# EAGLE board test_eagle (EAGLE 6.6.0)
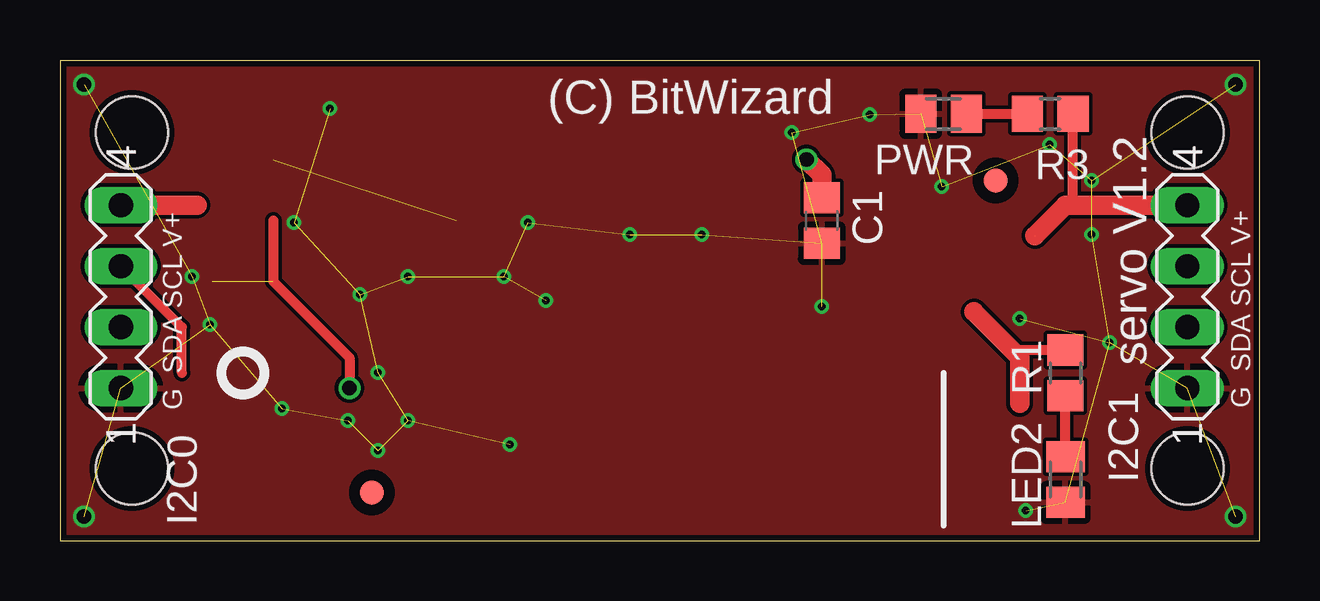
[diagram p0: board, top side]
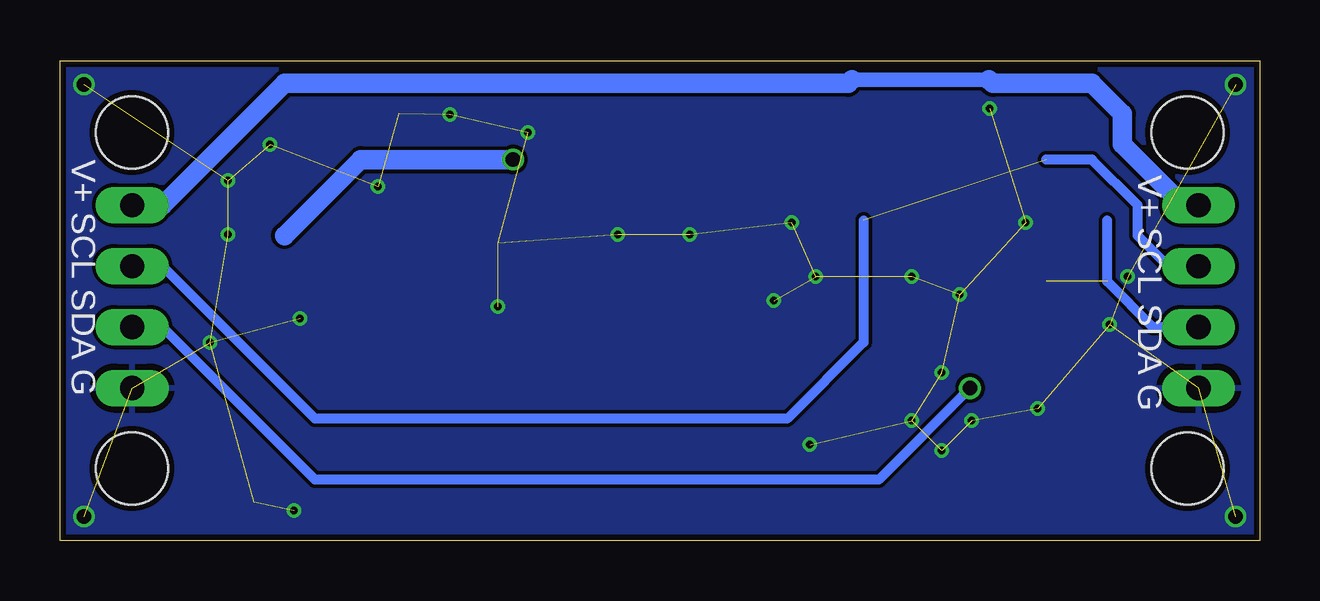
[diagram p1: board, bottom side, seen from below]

Size 50 x 20 mm. Coordinates in mm from the lower left corner, seen from the top.
Outline: 0,0 50,0 50,20 0,20 0,0
Copper layers (1*16): Top 0.035mm / dielectric 1.5mm / Bottom 0.035mm
Design rules "Fusion_eagle_rule_v1.1": minimum track width 6mil, minimum drill 12mil, track to track 6mil, track to pad 6mil, pad to pad 6mil, via to via 6mil, smd to smd 0mil, copper to edge 10mil, drill to drill 10mil, minimum pad ring 7mil, minimum via ring 6mil, stop-mask expansion 2mil, vias tented up to drill 100mil, thermal gap 10mil

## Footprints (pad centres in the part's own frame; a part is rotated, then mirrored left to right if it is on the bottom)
FID1 = smd 1 x 1: P$1 0,0
C0805 = smd 1.3 x 1.5: 1 -0.95,0; 2 0.95,0
MA04-1 = drill 1.016 long: 1 -3.81,0; 2 -1.27,0; 3 1.27,0; 4 3.81,0
M0805 = smd 1.3 x 1.6: 1 -0.95,0; 2 0.95,0
R0805 = smd 1.3 x 1.5: 1 -0.95,0; 2 0.95,0
MOUNTING_HOLE = hole 3: 0,0

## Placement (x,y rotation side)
AFIT1  FIDUCIAL1  [FID1]  13,2 0 top
AFIT2  FIDUCIAL1  [FID1]  39,15 0 top
C1  100n  [C0805]  31.75,13.34 270 top
I2C0  [MA04-1]  2.54,10.16 90 top
I2C1  [MA04-1]  46.99,10.16 90 top
LED2  G  [M0805]  41.91,2.54 270 top
PWR  G  [M0805]  36.83,17.78 180 top
R1  47k  [R0805]  41.91,6.99 90 top
R3  47k  [R0805]  41.27,17.78 0 top
U$2  MOUNTING_HOLE  [MOUNTING_HOLE]  3,3 0 top
U$3  MOUNTING_HOLE  [MOUNTING_HOLE]  3,17 0 top
U$4  MOUNTING_HOLE  [MOUNTING_HOLE]  47,3 0 top
U$5  MOUNTING_HOLE  [MOUNTING_HOLE]  47,17 0 top

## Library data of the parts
AFIT1 AFIT2 U$2-U$5 = hdr_altera
C1 R1 R3 = rcl
I2C0 I2C1 = con-lstb; OC_FARNELL: unknown; OC_NEWARK: unknown
LED2 PWR = myled

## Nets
GND: C1.2 I2C0.1 I2C1.1 LED2.2 PWR.2
N$1: I2C0.2 I2C1.2
N$6: PWR.1 R3.1
N$13: I2C0.3 I2C1.3
N$14: R1.2
N$15: LED2.1 R1.1
VCC: C1.1 I2C0.4 I2C1.4 R3.2

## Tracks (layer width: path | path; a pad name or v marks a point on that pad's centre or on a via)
GND  (via drill 0.3, 0.61)  (35 unrouted)
  other vias: 1,19 1,1 49,1 49,19 12,5 13.25,3.75 14.5,5 13.25,7 9.25,5.5 12.5,10.25 19.5,13.25 20.25,10 18.5,11 23.75,12.75 26.75,12.75 11.25,18 5.5,11 6.25,9 14.5,11 9.75,13.25 18.75,4 31.75,9.75 30.5,17 33.75,17.75 36.75,14.75 41.25,16.5 43,15 43,12.75 40.25,1.25 43.75,8.25 40,9.25
  pour Top: 0,20 0,0 50,0 50,20
  pour Bottom: 0,20 50,20 50,0 0,0
N$1  (via drill 0.61)  (1 unrouted)
  Top 0.406: 8.89,13.34 8.89,10.79 12.06,7.62 v12.06,6.35
  Bottom 0.406: I2C0.2 4.45,8.89 6.35,10.79 6.35,13.34 | v12.06,6.35 15.88,2.54 39.37,2.54 45.72,8.89 I2C1.2
N$6
  Top 0.406: PWR.1 R3.1
N$13  (1 unrouted)
  Top 0.406: 5.08,6.99 5.08,8.89 I2C0.3
  Bottom 0.406: 16.51,13.34 16.51,8.26 19.68,5.08 39.37,5.08 45.72,11.43 I2C1.3 | I2C0.3 3.81,11.43 5.08,12.7 5.08,13.97 6.99,15.88 8.89,15.88
N$14
  Top 0.406: R1.2 40.01,7.93 40.01,7.62
  Top 0.813: 40.01,5.71 40.01,7.62 38.1,9.53
N$15
  Top 0.406: LED2.1 R1.1
VCC  (via drill 0.61)  (1 unrouted)
  Top 0.406: v31.11,15.88 31.05,15.94 | 42.23,13.97 R3.2
  Top 0.813: v31.11,15.88 31.75,15.24 C1.1 32.07,14.29 | 5.71,13.97 I2C0.4 | I2C1.4 44.45,13.97 42.23,13.97 41.91,13.97 40.64,12.7
  Bottom 0.61: 11.27,19.21 16.99,19.21
  Bottom 0.813: v31.11,15.88 37.47,15.88 40.64,12.7 | I2C0.4 3.17,13.97 5.71,16.51 5.71,17.78 6.99,19.05 11.11,19.05 11.27,19.21 | I2C1.4 45.72,13.97 40.64,19.05 17.14,19.05 16.99,19.21

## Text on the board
tPlace: (C) BitWizard | servo V1.2 | G SDA SCL V+ | G SDA SCL V+
bPlace: V+ SCL SDA G | V+ SCL SDA G
tNames: I2C1 | I2C0
_tNames: PWR | IC1 | C1 | R3 | SV2 | SPI1 | SPI0 | SV1 | R1 | LED2
_bNames: SJ1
